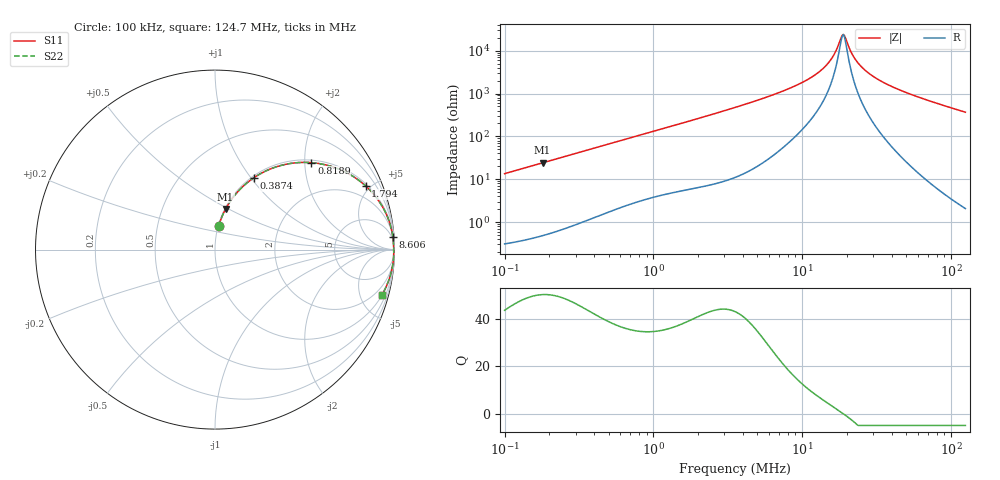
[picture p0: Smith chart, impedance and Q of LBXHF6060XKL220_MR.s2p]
! LBXHF6060XKL220_MR  S-PARAMETER MODEL  ( General Type )
! Model Generated by TAIYO YUDEN Corporation (http://www.ty-top.com)
! Version 1.0
! TAIYO YUDEN Control No. 220210
! Copyright(c) 2022 TAIYO YUDEN CO.,LTD. All Rights Reserved.
! Product Description (link to TY-COMPAS)
! https://ds.yuden.co.jp/TYCOMPAS/or/detail?pn=LBXHF6060XKL220MMR&u=M
! Products Name : Inductors
! Characteristics :
!  Inductance : 22 uH , SRF(min) : 15 MHz , DC Resistance(max) : 0.15 Ohm
!  Rated Current : Saturation :1500 mA , Temp Rise : 1900 mA
!  Case Size : 6.0 x 6.0 / 0.236 x 0.236 [mm/inch] , Thickness : 3 / 0.118 [mm/inch]
!  (Conditions: Temperature = 25 degC , DC Bias Current/Voltage = 0A / 0V)
! External Node Assignments :
!  1  o---GGG---o  2
! GND o---------o GND
! Frequency Range : 0.1MHz  -  124.6553MHz  [ 402 STEP ]
# MHz S RI R 50
! Freq[MHz].  S11 Real  S11 Imag  S21 Real  S21 Imag  S12 Real  S12 Imag  S22 Real  S22 Imag
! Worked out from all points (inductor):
!   401 points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, 100 kHz to 124.7 MHz, reference 50 ohm
!   read as one part in series: L = 21.4 uH near 103.6 kHz
!   highest Q = 50.2 at 180.1 kHz (marker M1), where L = 21.4 uH
!   self-resonance near 18.52 MHz
!   S11 on the Smith chart (normalised r, x): 100 kHz: 1.01, +0.27; 387.4 kHz: 1.02, +1.03; 818.9 kHz: 1.06, +2.16; 1.794 MHz: 1.12, +4.68; 8.606 MHz: 3, +28; 124.7 MHz: 1.04, -7.32
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0.1  0.0207 0.1315  0.9793 -0.1315  0.9793 -0.1315  0.0207 0.1315
0.180051  0.0592 0.2263  0.9408 -0.2263  0.9408 -0.2263  0.0592 0.2263
0.330013  0.1684 0.3633  0.8316 -0.3633  0.8316 -0.3633  0.1684 0.3633
0.387423  0.2164 0.4002  0.7836 -0.4002  0.7836 -0.4002  0.2164 0.4002
0.818907  0.5367 0.4844  0.4633 -0.4844  0.4633 -0.4844  0.5367 0.4844
1.089088  0.6662 0.4575  0.3338 -0.4575  0.3338 -0.4575  0.6662 0.4575
1.793754  0.8396 0.3546  0.1604 -0.3546  0.1604 -0.3546  0.8396 0.3546
3.530656  0.9528 0.2007  0.0472 -0.2007  0.0472 -0.2007  0.9528 0.2007
8.606354  0.9909 0.0695  0.00915 -0.0695  0.00915 -0.0695  0.9909 0.0695
11.65164  0.9939 0.0401  0.00607 -0.0401  0.00607 -0.0401  0.9939 0.0401
13.43696  0.9948 0.0277  0.00522 -0.0277  0.00522 -0.0277  0.9948 0.0277
15.22215  0.9953 0.0173  0.0047 -0.0173  0.0047 -0.0173  0.9953 0.0173
16.64073  0.9956 0.00998  0.00442 -0.00998  0.00442 -0.00998  0.9956 0.00998
18.19151  0.9958 0.00276  0.00423 -0.00276  0.00423 -0.00276  0.9958 0.00276
18.85157  0.9958 -0.000122  0.00417 0.000122  0.00417 0.000122  0.9958 -0.000122
19.53556  0.9959 -0.00301  0.00413 0.00301  0.00413 0.00301  0.9959 -0.00301
22.13099  0.9959 -0.0132  0.00408 0.0132  0.00408 0.0132  0.9959 -0.0132
24.62842  0.9958 -0.0222  0.00419 0.0222  0.00419 0.0222  0.9958 -0.0222
29.43265  0.9952 -0.0378  0.00475 0.0378  0.00475 0.0378  0.9952 -0.0378
38.45196  0.9931 -0.0639  0.00687 0.0639  0.00687 0.0639  0.9931 -0.0639
63.33127  0.9818 -0.1261  0.0182 0.1261  0.0182 0.1261  0.9818 -0.1261
124.6553  0.9293 -0.2535  0.0707 0.2535  0.0707 0.2535  0.9293 -0.2535
